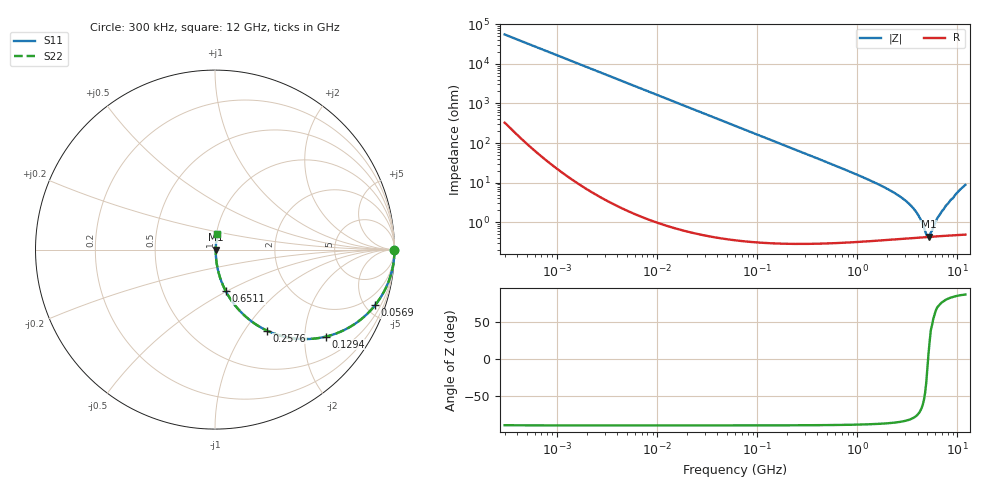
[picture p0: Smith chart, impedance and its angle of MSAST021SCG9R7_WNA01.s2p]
! MSAST021SCG9R7_WNA01  S-PARAMETER MODEL  ( General Type )
! Model Generated by TAIYO YUDEN Corporation (http://www.ty-top.com)
! Version 2.0
! TAIYO YUDEN Control No. 181101
! Copyright(c) 2015 TAIYO YUDEN CO.,LTD. All Rights Reserved.
! Product Description (link to TY-COMPAS)
! https://ds.yuden.co.jp/TYCOMPAS/or/detail?pn=MSAST021SCG9R7CWNA01&u=M
! Products Name : Multilayer Ceramic Capacitors
! Characteristics :
!  Capacitance : 9.7 pF , Rated Voltage : 25V , TCC : CG / C0G
!  Case Size : 0.25 x 0.125 / 0.0098 x 0.0049 [mm/inch] , Thickness : 0.125 / 0.0049 [mm/inch]
!  (Conditions: Temperature = 25 degC , DC Bias Current/Voltage = 0A / 0V)
! External Node Assignments :
!  1  o---| |---o  2
! GND o---------o GND
! Frequency Range : 0.3MHz  -  12000MHz  [ 401 STEP ]
# MHz S RI R 50
! Freq[MHz].  S11 Real  S11 Imag  S21 Real  S21 Imag  S12 Real  S12 Imag  S22 Real  S22 Imag
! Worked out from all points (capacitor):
!   401 points, 300 kHz to 12 GHz, reference 50 ohm
!   read as one part in series: C = 9.7 pF near 316.3 kHz
!   lowest |Z| = 431 mohm at 5.141 GHz (marker M1)
!   series resonance near 5.093 GHz, so ESL is about 100 pH
!   S11 on the Smith chart (normalised r, x): 300 kHz: open; 56.9 MHz: 1.01, -5.77; 129.4 MHz: 1.01, -2.54; 257.6 MHz: 1.01, -1.27; 651.1 MHz: 1.01, -0.50; 12 GHz: 1.01, +0.18
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0.3  1 -0.00183  1.42e-05 0.00183  1.42e-05 0.00183  1 -0.00183
1.769972  0.9999 -0.0108  0.000126 0.0108  0.000126 0.0108  0.9999 -0.0108
10.44266  0.9959 -0.0634  0.00407 0.0634  0.00407 0.0634  0.9959 -0.0634
25.70316  0.9759 -0.1529  0.0241 0.1529  0.0241 0.1529  0.9759 -0.1529
56.90376  0.8923 -0.3094  0.1077 0.3094  0.1077 0.3094  0.8923 -0.3094
60  0.8817 -0.3223  0.1183 0.3223  0.1183 0.3223  0.8817 -0.3223
129.3602  0.6161 -0.4852  0.3839 0.4852  0.3839 0.4852  0.6161 -0.4852
182.544  0.4464 -0.4955  0.5536 0.4955  0.5536 0.4955  0.4464 -0.4955
257.5933  0.2884 -0.4508  0.7116 0.4508  0.7116 0.4508  0.2884 -0.4508
353.9943  0.177 -0.3785  0.823 0.3785  0.823 0.3785  0.177 -0.3785
651.0506  0.0604 -0.2322  0.9396 0.2322  0.9396 0.2322  0.0604 -0.2322
2088.533  0.0078 -0.0646  0.9922 0.0646  0.9922 0.0646  0.0078 -0.0646
2870.14  0.00532 -0.0386  0.9947 0.0386  0.9947 0.0386  0.00532 -0.0386
3547.679  0.00453 -0.0235  0.9955 0.0235  0.9955 0.0235  0.00453 -0.0235
4050.141  0.00429 -0.0147  0.9957 0.0147  0.9957 0.0147  0.00429 -0.0147
4875.354  0.00422 -0.00267  0.9958 0.00267  0.9958 0.00267  0.00422 -0.00267
5140.631  0.00426 0.000532  0.9957 -0.000532  0.9957 -0.000532  0.00426 0.000532
5420.343  0.00431 0.00345  0.9957 -0.00345  0.9957 -0.00345  0.00431 0.00345
6354.153  0.00457 0.0124  0.9954 -0.0124  0.9954 -0.0124  0.00457 0.0124
7254.098  0.00494 0.0205  0.9951 -0.0205  0.9951 -0.0205  0.00494 0.0205
9968.853  0.00783 0.0554  0.9922 -0.0554  0.9922 -0.0554  0.00783 0.0554
12000  0.0124 0.0862  0.9876 -0.0862  0.9876 -0.0862  0.0124 0.0862
